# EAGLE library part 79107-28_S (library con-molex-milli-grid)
RECEPTACAL
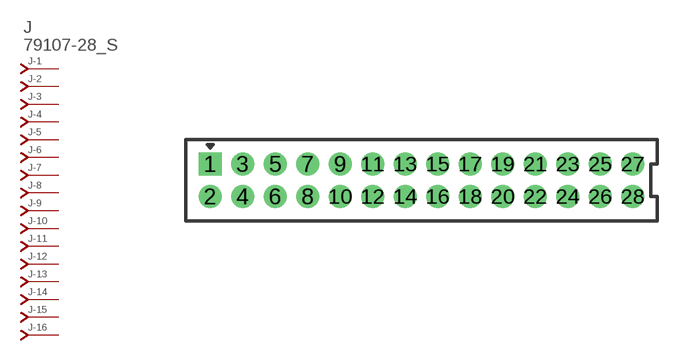
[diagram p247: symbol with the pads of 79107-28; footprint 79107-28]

Designator prefix J; gates -1=J-NV -2=J-N -3=J-N -4=J-N -5=J-N -6=J-N -7=J-N -8=J-N -9=J-N -10=J-N -11=J-N -12=J-N -13=J-N -14=J-N -15=J-N -16=J-N -17=J-N -18=J-N -19=J-N -20=J-N -21=J-N -22=J-N -23=J-N -24=J-N -25=J-N -26=J-N -27=J-N -28=J-N

## 79107-28_S  [79107-28]
1  -1:J  pas
2  -2:J  pas
3  -3:J  pas
4  -4:J  pas
5  -5:J  pas
6  -6:J  pas
7  -7:J  pas
8  -8:J  pas
9  -9:J  pas
10  -10:J  pas
11  -11:J  pas
12  -12:J  pas
13  -13:J  pas
14  -14:J  pas
15  -15:J  pas
16  -16:J  pas
17  -17:J  pas
18  -18:J  pas
19  -19:J  pas
20  -20:J  pas
21  -21:J  pas
22  -22:J  pas
23  -23:J  pas
24  -24:J  pas
25  -25:J  pas
26  -26:J  pas
27  -27:J  pas
28  -28:J  pas

## Footprint 79107-28 (pad centres in mm)
RECEPTACAL Dual Row, Vertical, Through-Hole
drill 0.914 square: 1 -13,1
drill 0.914: 2 -13,-1; 3 -11,1; 4 -11,-1; 5 -9,1; 6 -9,-1; 7 -7,1; 8 -7,-1; 9 -5,1; 10 -5,-1; 11 -3,1; 12 -3,-1; 13 -1,1; 14 -1,-1; 15 1,1; 16 1,-1; 17 3,1; 18 3,-1; 19 5,1; 20 5,-1; 21 7,1; 22 7,-1; 23 9,1; 24 9,-1; 25 11,1; 26 11,-1; 27 13,1; 28 13,-1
